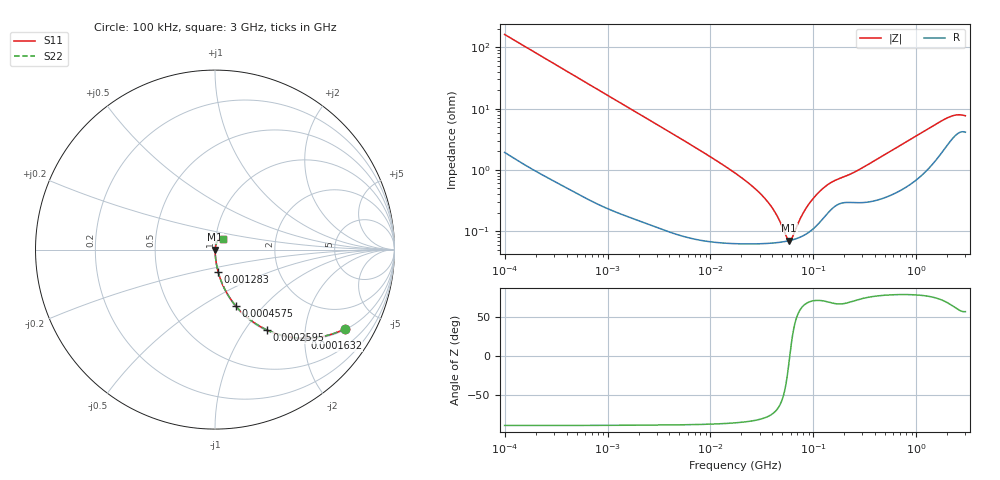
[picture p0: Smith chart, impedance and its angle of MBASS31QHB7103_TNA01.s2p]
! MBASS31QHB7103_TNA01  S-PARAMETER MODEL  ( Standard Model )
! Model Generated by TAIYO YUDEN Corporation (http://www.ty-top.com)
! Version 2.0
! TAIYO YUDEN Control No. 231201
! Copyright(c) 2013 TAIYO YUDEN CO.,LTD. All Rights Reserved.
! Product Description (link to TY-COMPAS)
! https://ds.yuden.co.jp/TYCOMPAS/or/detail?pn=MBASS31QHB7103KTNA01&u=M
! Products Name : Multilayer Ceramic Capacitors
! Characteristics :
!  Capacitance : 0.01 [uF] , Rated Voltage : 630 [V] , TCC : X7R
!  Case Size : 3.2 x 1.6 / 0.126 x 0.063 [mm/inch] , Thickness : 1.15 / 0.045 [mm/inch]
!  (Conditions: Temperature = 25 [degC] , DC Bias Voltage = 0 [V])
! External Node Assignments :
!  1  o---| |---o  2
! GND o---------o GND
! Frequency Range : 100kHz  -  3GHz  [ 401 STEP ]
# MHZ S RI R 50
! Freq[MHz].  S11 Real  S11 Imag  S21 Real  S21 Imag  S12 Real  S12 Imag  S22 Real  S22 Imag
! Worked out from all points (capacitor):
!   401 points, 100 kHz to 3 GHz, reference 50 ohm
!   read as one part in series: C = 9.76 nF near 105.3 kHz
!   lowest |Z| = 70.1 mohm at 58.16 MHz (marker M1)
!   series resonance near 58.98 MHz, so ESL is about 750 pH
!   S11 on the Smith chart (normalised r, x): 100 kHz: 1.04, -3.25; 163.2 kHz: 1.02, -2.00; 259.5 kHz: 1.01, -1.26; 457.5 kHz: 1.01, -0.72; 1.283 MHz: 1.00, -0.26; 3 GHz: 1.08, +0.13
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0.1  0.7234 -0.4414  0.2766 0.4414  0.2766 0.4414  0.7234 -0.4414
0.163179  0.5002 -0.4942  0.4998 0.4942  0.4998 0.4942  0.5002 -0.4942
0.259498  0.2871 -0.4465  0.7129 0.4465  0.7129 0.4465  0.2871 -0.4465
0.457483  0.1174 -0.3157  0.8826 0.3157  0.8826 0.3157  0.1174 -0.3157
0.562235  0.0818 -0.2678  0.9182 0.2678  0.9182 0.2678  0.0818 -0.2678
1.282589  0.0182 -0.1264  0.9818 0.1264  0.9818 0.1264  0.0182 -0.1264
3.161081  0.00386 -0.0523  0.9961 0.0523  0.9961 0.0523  0.00386 -0.0523
17.7727  0.000695 -0.00859  0.9993 0.00859  0.9993 0.00859  0.000695 -0.00859
26.84345  0.000642 -0.00497  0.9994 0.00497  0.9994 0.00497  0.000642 -0.00497
35.64176  0.000637 -0.00301  0.9994 0.00301  0.9994 0.00301  0.000637 -0.00301
42.68829  0.000646 -0.00189  0.9994 0.00189  0.9994 0.00189  0.000646 -0.00189
53.83243  0.000678 -0.000527  0.9993 0.000527  0.9993 0.000527  0.000678 -0.000527
58.15973  0.000696 -8.03e-05  0.9993 8.03e-05  0.9993 8.03e-05  0.000696 -8.03e-05
62.83488  0.000719 0.000368  0.9993 -0.000368  0.9993 -0.000368  0.000719 0.000368
79.23846  0.000838 0.00175  0.9992 -0.00175  0.9992 -0.00175  0.000838 0.00175
97.38194  0.00106 0.00308  0.9989 -0.00308  0.9989 -0.00308  0.00106 0.00308
147.0833  0.00223 0.00573  0.9978 -0.00573  0.9978 -0.00573  0.00223 0.00573
259.3015  0.00298 0.00895  0.997 -0.00895  0.997 -0.00895  0.00298 0.00895
547.5153  0.00411 0.0191  0.9959 -0.0191  0.9959 -0.0191  0.00411 0.0191
1935.725  0.0268 0.0614  0.9732 -0.0614  0.9732 -0.0614  0.0268 0.0614
2441.062  0.0403 0.0642  0.9597 -0.0642  0.9597 -0.0642  0.0403 0.0642
3000  0.0432 0.0593  0.9568 -0.0593  0.9568 -0.0593  0.0432 0.0593
